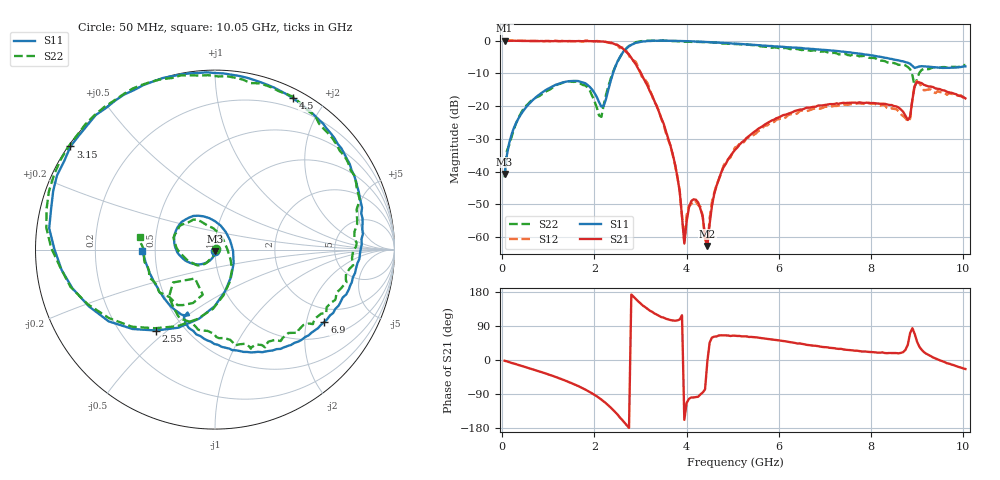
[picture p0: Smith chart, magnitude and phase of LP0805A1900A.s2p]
! AVX THIN FILM OPERATION
! 0805 Size Low Pass Filter P/N  LP0805A1900AWTR
! Network Analyzer HP8720ES.07.64: Feb 23, 2000 Serial No. US39172382
! Hewlett-Packard
!  2 Feb 2003  04:16:59
! Frequency  S11  S21  S12  S22
# HZ  S  DB R  50
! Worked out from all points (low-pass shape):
!   201 points, 50 MHz to 10.05 GHz, reference 50 ohm
!   highest |S21| = 0.00 dB at 50 MHz (marker M1); lowest = -62.7 dB at 4.45 GHz (marker M2)
!   |S21| within 3 dB of the highest: start of sweep to 2.662 GHz
!   lowest |S11| = -40.8 dB at 50 MHz (marker M3), VSWR 1.02, Z = 50.1 - j0.914 ohm
!   |S11| at or under -10 dB: start of sweep to 2.401 GHz
!   |S22| runs from -41.8 to 0.1 dB; largest |S21 - S12| = 0.066
!   S11 on the Smith chart (normalised r, x): 50 MHz: 1.00, -0.02; 2.55 GHz: 0.35, -0.46; 3.15 GHz: 0.01, +0.32; 4.5 GHz: 0.10, +1.63; 6.9 GHz: 1.49, -2.56; 10.05 GHz: 0.42, -0.01
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5e7  -40.77 -85.3  -0.00 -2.0  0.01 -2.0  -41.76 14.8
1e8  -34.93 -93.5  -0.03 -3.6  -0.01 -3.8  -33.68 -94.0
5e8  -20.62 -126.0  -0.08 -18.6  -0.06 -18.9  -20.12 -126.0
1.75e9  -12.78 129.3  -0.14 -74.8  -0.25 -75.1  -13.54 132.7
2.15e9  -20.13 31.4  -0.23 -104.5  -0.24 -105.0  -23.28 2.8
2.55e9  -5.08 -126.0  -1.80 -151.5  -2.25 -151.4  -5.17 -127.4
2.85e9  -0.96 179.7  -6.30 166.9  -6.04 171.2  -0.79 179.4
3.15e9  -0.09 144.5  -13.77 134.9  -12.96 132.0  -0.02 145.5
3.4e9  -0.01 123.8  -21.75 116.7  -21.58 112.1  0.02 124.2
3.75e9  -0.05 101.0  -37.84 103.8  -38.06 104.5  -0.10 101.1
3.95e9  -0.14 90.0  -62.00 -157.9  -61.35 -161.1  -0.31 88.8
4.15e9  -0.23 79.6  -48.48 -98.8  -48.83 -98.8  -0.45 77.9
4.45e9  -0.42 65.1  -62.70 -3.9  -62.80 11.5  -0.39 63.0
4.5e9  -0.46 62.8  -55.99 46.0  -54.25 53.4  -0.45 61.2
4.65e9  -0.56 55.9  -44.32 62.2  -43.98 58.1  -0.62 54.5
5.05e9  -0.89 38.6  -33.36 64.1  -32.66 60.9  -1.02 36.1
6.75e9  -2.53 -28.2  -20.22 37.8  -20.81 38.3  -2.93 -29.7
6.9e9  -2.73 -33.4  -19.79 35.1  -20.78 35.3  -3.37 -34.1
8.4e9  -5.50 -88.2  -19.65 18.5  -20.87 17.3  -6.84 -95.2
8.8e9  -6.74 -108.5  -24.24 40.2  -24.70 40.2  -8.04 -125.7
9e9  -8.11 -111.6  -12.70 48.7  -12.42 40.1  -11.70 -105.2
1.005e10  -7.85 -179.3  -17.62 -23.7  -17.36 -19.0  -7.43 170.6
